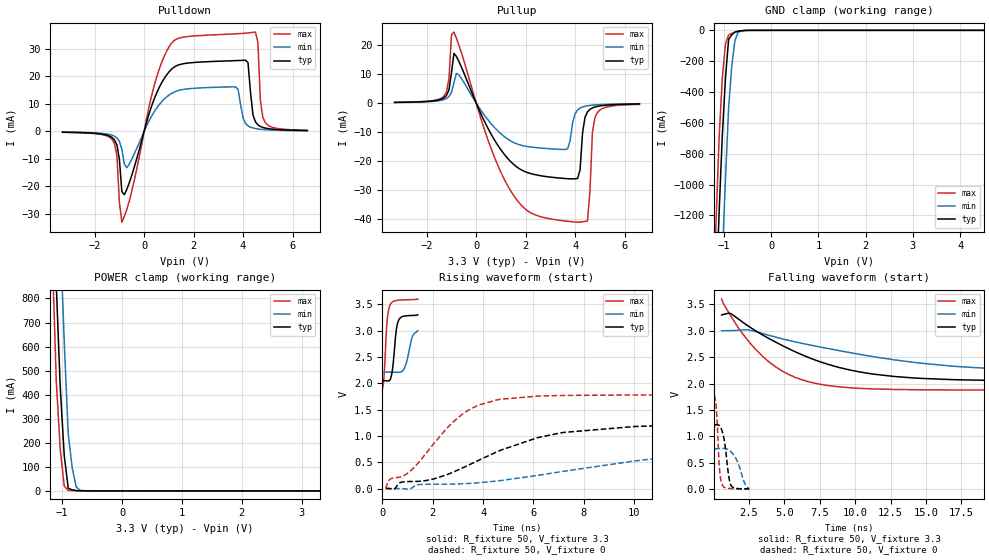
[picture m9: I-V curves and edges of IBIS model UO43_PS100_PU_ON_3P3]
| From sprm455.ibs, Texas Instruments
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|   Model Cell UO43_PS100_PU_ON_3P3
|IDG09_OUO43_PS100_PU_ON_3P3
[Model]   UO43_PS100_PU_ON_3P3
Model_type   I/O
Polarity   Non-Inverting
Enable   Active-Low
Vinl =  0.8V
Vinh =  2V
Cref =  15pF
Rref =  100.00M
Vref =  0V
Vmeas =  1.65
C_comp   1.7423p   1.5272001p   2.1795998p
[Model Spec]
Vinl   0.8V   0.8V   0.8V
Vinh   2V   2V   2V
[Temperature Range]   25   125   -40
[Voltage Range]   3.3   3   3.6
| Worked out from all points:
|   slope of the pulldown table from 0 to 0.495 V, typ, clamps not added: 36.1 ohm
|   slope of the pullup table from 0 to 0.495 V, typ, clamps not added: 54.7 ohm
|   GND clamp passes 1 mA (typ) near -0.56 V on its own axis
|   POWER clamp passes 1 mA (typ) near -0.77 V on its own axis
|   rising waveform, R_fixture 50, V_fixture 3.3: 20-80 % time 155ps typ, 223ps min, 126ps max; typ from 2.05 V to 3.3 V
|   rising waveform, R_fixture 50, V_fixture 0: 20-80 % time 3.76ns typ, 7.18ns min, 2.05ns max; typ from 0.002 V to 1.21 V
|   falling waveform, R_fixture 50, V_fixture 3.3: 20-80 % time 6.27ns typ, 10.3ns min, 3.67ns max; typ from 3.3 V to 2.05 V
|   falling waveform, R_fixture 50, V_fixture 0: 20-80 % time 343ps typ, 625ps min, 206ps max; typ from 1.21 V to 0.002 V
[POWER_clamp]
|   voltage   I(typ)   I(min)   I(max)
-3.3V     22.02A     22.67A     21.68A
-1.167V   1.409A     2.149A     988.2mA
-1.1V     858.4mA    1.581A     457.3mA
-1.033V   429.7mA    1.068A     171.9mA
-966.7mV  147.2mA    619.1mA    20.2mA
-900mV    11.07mA    235.7mA    2.195mA
-833.3mV  4.43mA     94.85mA    1.546mA
-766.7mV  907.1uA    16.91mA    1.026mA
-700mV    496.4uA    1.9mA      634.6uA
3.3V      -113.8uA   -75.38uA   -192.6uA
[Pulldown]
|   voltage   I(typ)   I(min)   I(max)
-3.3V     -317uA     -253.1uA   -342.7uA
-1.3V     -2.213mA   -1.382mA   -2.895mA
-1.1V     -4.939mA   -2.395mA   -8.797mA
-900mV    -21.96mA   -6.503mA   -33.05mA
-700mV    -21.08mA   -13.26mA   -28.39mA
1.1V      22.53mA    13.75mA    32mA
3.7V      25.73mA    16.16mA    35.48mA
4.1V      25.87mA    2.915mA    35.73mA
4.5V      3.469mA    1.015mA    36.11mA
4.7V      1.79mA     755.5uA    11.4mA
4.9V      1.19mA     600.1uA    3.153mA
6.6V      301uA      215.6uA    389.3uA
[Pullup]
|   voltage   I(typ)   I(min)   I(max)
-3.3V     241.9uA    204.6uA    268.8uA
-1.3V     1.834mA    1.218mA    2.447mA
-900mV    17.22mA    7.132mA    24.6mA
500mV     -9.137mA   -6.074mA   -13.34mA
1.5V      -21.13mA   -13.59mA   -31.83mA
3.7V      -26.2mA    -15.82mA   -40.94mA
4.1V      -26.12mA   -2.383mA   -41.26mA
4.5V      -3.039mA   -932.7uA   -40.81mA
4.6V      -2.168mA   -805.3uA   -30.42mA
4.7V      -1.674mA   -708uA     -10.08mA
4.9V      -1.143mA   -569.3uA   -3.269mA
6.6V      -301.8uA   -211.1uA   -437.5uA
[GND_clamp]
|   voltage   I(typ)   I(min)   I(max)
-3.3V     -22.41A    -23.18A    -21.98A
-1.233V   -2.33A     -3.195A    -1.825A
-1.167V   -1.743A    -2.601A    -1.246A
-1.1V     -1.172A    -2.017A    -690.4mA
-1.033V   -681.5mA   -1.471A    -309.1mA
-966.7mV  -310.3mA   -965.9mA   -88.82mA
-900mV    -58.4mA    -501.8mA   -29.5mA
-833.3mV  -28.81mA   -231.8mA   -20.35mA
-766.7mV  -11.28mA   -68.53mA   -12.51mA
-700mV    -5.803mA   -11.89mA   -5.973mA
-500mV    -272.6uA   -567.4uA   -249.8uA
6.6V      0A         0A         0A
[Ramp]
| variable   typ   min   max
dV/dt_f 0.76841966/6.3089267n 0.48404526/10.391204n  1.0587507/3.6908192n
dV/dt_r 0.73311356/3.7813818n 0.46426152/7.1680451n  1.0737974/2.0631676n
R_load = 50
[Rising Waveform]
R_fixture = 50
V_fixture = 3.3
V_fixture_min = 3
V_fixture_max = 3.6
|   time   V(typ)   V(min)   V(max)
0s        2.05V      2.213V     1.878V
72.92ps   2.05V      2.213V     2.182V
186.7ps   2.046V     2.214V     3.174V
288.8ps   2.057V     2.213V     3.467V
394.6ps   2.242V     2.212V     3.544V
543.6ps   2.975V     2.21V      3.572V
640.5ps   3.19V      2.208V     3.579V
886.5ps   3.278V     2.3V       3.585V
1.182ns   3.289V     2.872V     3.59V
1.406ns   3.3V       3V         3.6V
[Rising Waveform]
R_fixture = 50
V_fixture = 0
V_fixture_min = 0
V_fixture_max = 0
|   time   V(typ)   V(min)   V(max)
141.5ps   2.058mV    1.645mV    2.758mV
320.7ps   -1.912mV   1.801mV    181.5mV
746.1ps   120.1mV    655.1uV    225.3mV
1.146ns   135.1mV    6.599mV    349.4mV
2.019ns   181.3mV    83.17mV    842mV
3.115ns   377.8mV    90.39mV    1.391V
4.542ns   697.4mV    144.7mV    1.684V
7.174ns   1.067V     327.5mV    1.77V
10.04ns   1.181V     527.1mV    1.778V
18.76ns   1.211V     765.4mV    1.779V
[Falling Waveform]
R_fixture = 50
V_fixture = 3.3
V_fixture_min = 3
V_fixture_max = 3.6
|   time   V(typ)   V(min)   V(max)
581.5ps   3.3V       3V         3.6V
1.232ns   3.325V     3.003V     3.281V
2.286ns   3.122V     3.019V     2.867V
3.492ns   2.918V     2.947V     2.512V
4.876ns   2.719V     2.846V     2.235V
6.641ns   2.502V     2.741V     2.041V
9.63ns    2.257V     2.586V     1.921V
12.73ns   2.135V     2.451V     1.889V
17.64ns   2.07V      2.316V     1.88V
25.58ns   2.05V      2.213V     1.878V
[Falling Waveform]
R_fixture = 50
V_fixture = 0
V_fixture_min = 0
V_fixture_max = 0
|   time   V(typ)   V(min)   V(max)
74.75ps   1.211V     765.4mV    1.779V
225.3ps   1.221V     766.1mV    1.464V
439.6ps   1.2V       770.7mV    362.3mV
600.2ps   1.115V     773.3mV    101.7mV
765.6ps   932.4mV    772.2mV    36.49mV
1.081ns   248.3mV    742.8mV    15.13mV
1.217ns   87.55mV    715mV      13mV
1.66ns    14.25mV    544.8mV    8.345mV
2.201ns   8.153mV    118.7mV    5.636mV
2.516ns   2.058mV    1.645mV    2.758mV
